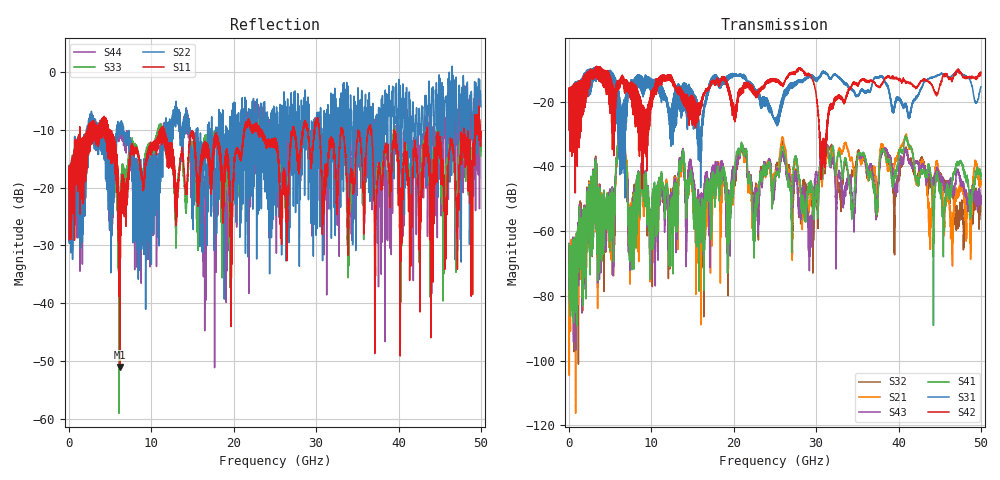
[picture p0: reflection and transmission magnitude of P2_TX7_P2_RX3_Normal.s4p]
!Keysight Technologies,N5225B,MY57041031,A.13.20.10
!Date: Friday, May 31, 2019 11:31:22
!Correction: S11(Full 4 Port(1,2,3,4))
!S12(Full 4 Port(1,2,3,4))
!S13(Full 4 Port(1,2,3,4))
!S14(Full 4 Port(1,2,3,4))
!S21(Full 4 Port(1,2,3,4))
!S22(Full 4 Port(1,2,3,4))
!S23(Full 4 Port(1,2,3,4))
!S24(Full 4 Port(1,2,3,4))
!S31(Full 4 Port(1,2,3,4))
!S32(Full 4 Port(1,2,3,4))
!S33(Full 4 Port(1,2,3,4))
!S34(Full 4 Port(1,2,3,4))
!S41(Full 4 Port(1,2,3,4))
!S42(Full 4 Port(1,2,3,4))
!S43(Full 4 Port(1,2,3,4))
!S44(Full 4 Port(1,2,3,4))
!S4P File: Measurements: <S11,S12,S13,S14>,
!<S21,S22,S23,S24>,
!<S31,S32,S33,S34>,
!<S41,S42,S43,S44>:
# Hz S  dB  R 50.0
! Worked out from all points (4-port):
!   5000 points, 10 MHz to 50 GHz, reference 50 ohm
!   strongest paths, dB at 10 MHz, 12.51 GHz, 25.01 GHz, 37.51 GHz, 50 GHz:
!     S42: -19.4, -14.2, -13.2, -15.3, -10.9
!     S31: -19.6, -22.0, -25.8, -12.8, -15.4
!     S41: -63.9, -50.8, -42.8, -47.6, -42.8
!     S43: -63.8, -49.2, -46.3, -49.1, -51.4
!     S21: -69.3, -48.4, -42.1, -47.1, -44.0
!     S32: -67.3, -47.1, -41.9, -47.3, -50.2
!   lowest |S11| = -51.1 dB at 6.19 GHz (marker M1), VSWR 1.01, Z = 50.2 + j0.193 ohm
!   |S11| at or under -10 dB: 4.911 GHz to 11.03 GHz (6.119 GHz wide, 76.8 % of centre); 11.57 GHz to 21.26 GHz (9.687 GHz wide, 59 % of centre); 43.5 GHz to 47.91 GHz (4.411 GHz wide, 9.65 % of centre)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
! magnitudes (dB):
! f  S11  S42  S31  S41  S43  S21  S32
! 10 MHz  -20.2  -19.4  -19.6  -63.9  -63.8  -69.3  -67.3
! 6.19 GHz  -51.1  -15.2  -19.6  -31.9  -31.1  -32.9  -32.1
! 7.45 GHz  -14.7  -14.4  -13.9  -54.4  -55.4  -53.7  -54.4
! 21.08 GHz  -12.8  -15.9  -12.4  -33.4  -33.5  -34.7  -34.3
! 28.08 GHz  -14.5  -9.8  -13.5  -46.7  -54.2  -48.6  -55.1
! 30.78 GHz  -20.6  -33.3  -10.9  -43.6  -40.2  -43.9  -41.2
! 50 GHz  -11.2  -10.9  -15.4  -42.8  -51.4  -44.0  -50.2
